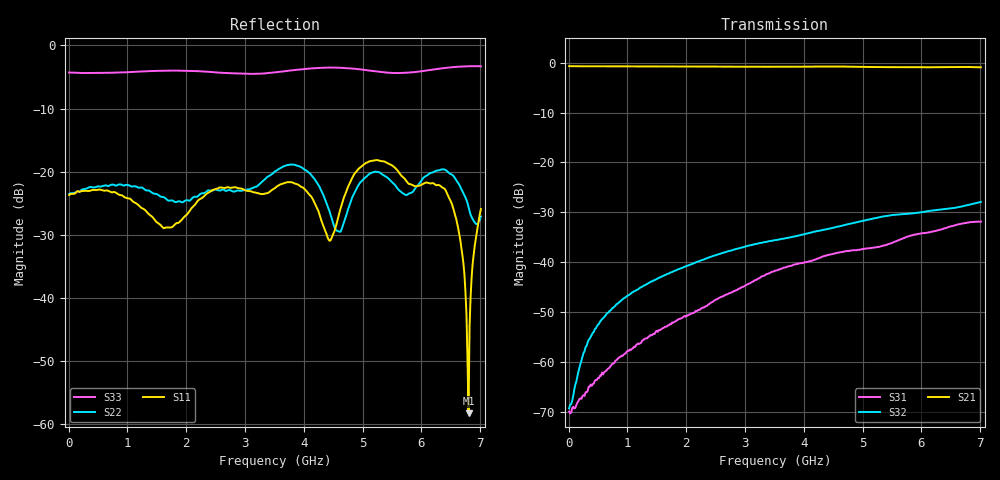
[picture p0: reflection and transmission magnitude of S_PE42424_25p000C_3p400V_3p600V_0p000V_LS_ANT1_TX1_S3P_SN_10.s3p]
! Device ID: PE42424
! Device ID: PE42424
! File Path: z:\PE42424\Characterization\RAW\25p000C\3p400\LS_ANT1_TX1\PE42424_25p000C_3p400V_3p600V_0p000V_LS_ANT1_TX1_S3P_SN_10_.s3p
! Serial: 10
! Lot:
! Temp: 25.000C
! VDD: 3.400
! VSS: 0.000
! Control_Hi: 3.600
! Control_Lo: 0.000
! Logic State: LS_ANT1_TX1
! Port 1: RFC
! Port 2: RF1
! Port 3: RF2
! ThroughPath:1-2
! IDD: 0.0001269841
! ISS: -1.719e-007
#  Hz  S  RI  R  50
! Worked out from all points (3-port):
!   401 points, 10 MHz to 7.01 GHz, reference 50 ohm
!   strongest paths, dB at 10 MHz, 1.76 GHz, 3.51 GHz, 5.26 GHz, 7.01 GHz:
!     S21: -0.7, -0.8, -0.8, -0.9, -1.0
!     S32: -69.2, -41.9, -35.5, -31.0, -27.9
!     S31: -69.9, -52.0, -41.7, -36.9, -31.8
!   lowest |S11| = -58.2 dB at 6.8 GHz (marker M1), VSWR 1.00, Z = 49.9 - j0.0507 ohm
!   |S11| at or under -10 dB: start of sweep to end of sweep
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1e7  0.0654 -0.000471  0.921 -0.00309  0.000333 -1.71e-05
     0.9195 -0.00349  0.0666 -0.000671  0.000326 0.000113
     0.000322 1.65e-06  0.000339 7.48e-05  -0.6103 0.00218
9.2e8  0.0623 0.0169  0.9056 -0.1381  -0.00101 -0.000578
       0.9053 -0.1378  0.0763 0.017  0.000579 0.00422
       -0.00101 -0.000564  0.000606 0.00423  -0.5907 0.1595
1.655e9  0.0351 -0.00889  0.8811 -0.2453  -0.00225 -0.000238
         0.8804 -0.2447  0.0609 -0.00634  0.000937 0.00748
         -0.00226 -0.000253  0.000962 0.00745  -0.5797 0.2497
3.51e9  0.0737 0.0092  0.7647 -0.4885  -0.00741 0.00355
        0.7645 -0.4898  0.1002 0.0107  0.00391 0.0162
        -0.00744 0.00355  0.00387 0.0162  -0.3763 0.4824
4.595e9  -0.000564 -0.0456  0.6671 -0.6216  -0.00871 0.00908
         0.6661 -0.6222  0.0193 -0.0277  0.00584 0.0222
         -0.00872 0.00906  0.00588 0.0221  -0.3535 0.5641
5.1375e9  -0.0447 -0.1131  0.6001 -0.6734  -0.00833 0.0111
          0.5991 -0.6746  -0.0395 -0.0893  0.00833 0.0258
          -0.00834 0.0111  0.00839 0.0258  -0.3012 0.5536
6.3625e9  0.0747 0.00122  0.4589 -0.7736  -0.00921 0.0196
          0.4577 -0.7733  0.1038 -0.0133  0.0149 0.0304
          -0.00906 0.0196  0.0151 0.0304  -0.0313 0.6583
6.6425e9  0.0311 0.00741  0.4198 -0.7983  -0.00815 0.0226
          0.4197 -0.7989  0.0764 -0.0198  0.0158 0.0321
          -0.00808 0.0227  0.016 0.0322  -0.0251 0.6785
6.8e9  -0.00111 -0.000508  0.3955 -0.8098  -0.00687 0.0242
       0.3943 -0.81  0.0443 -0.0283  0.0166 0.0336
       -0.00675 0.0241  0.0169 0.0337  -0.0281 0.6834
7.01e9  -0.0447 -0.0239  0.361 -0.8198  -0.00476 0.0251
        0.3606 -0.8195  -0.0114 -0.0427  0.0187 0.0357
        -0.00473 0.0251  0.0188 0.0357  -0.0345 0.6826
